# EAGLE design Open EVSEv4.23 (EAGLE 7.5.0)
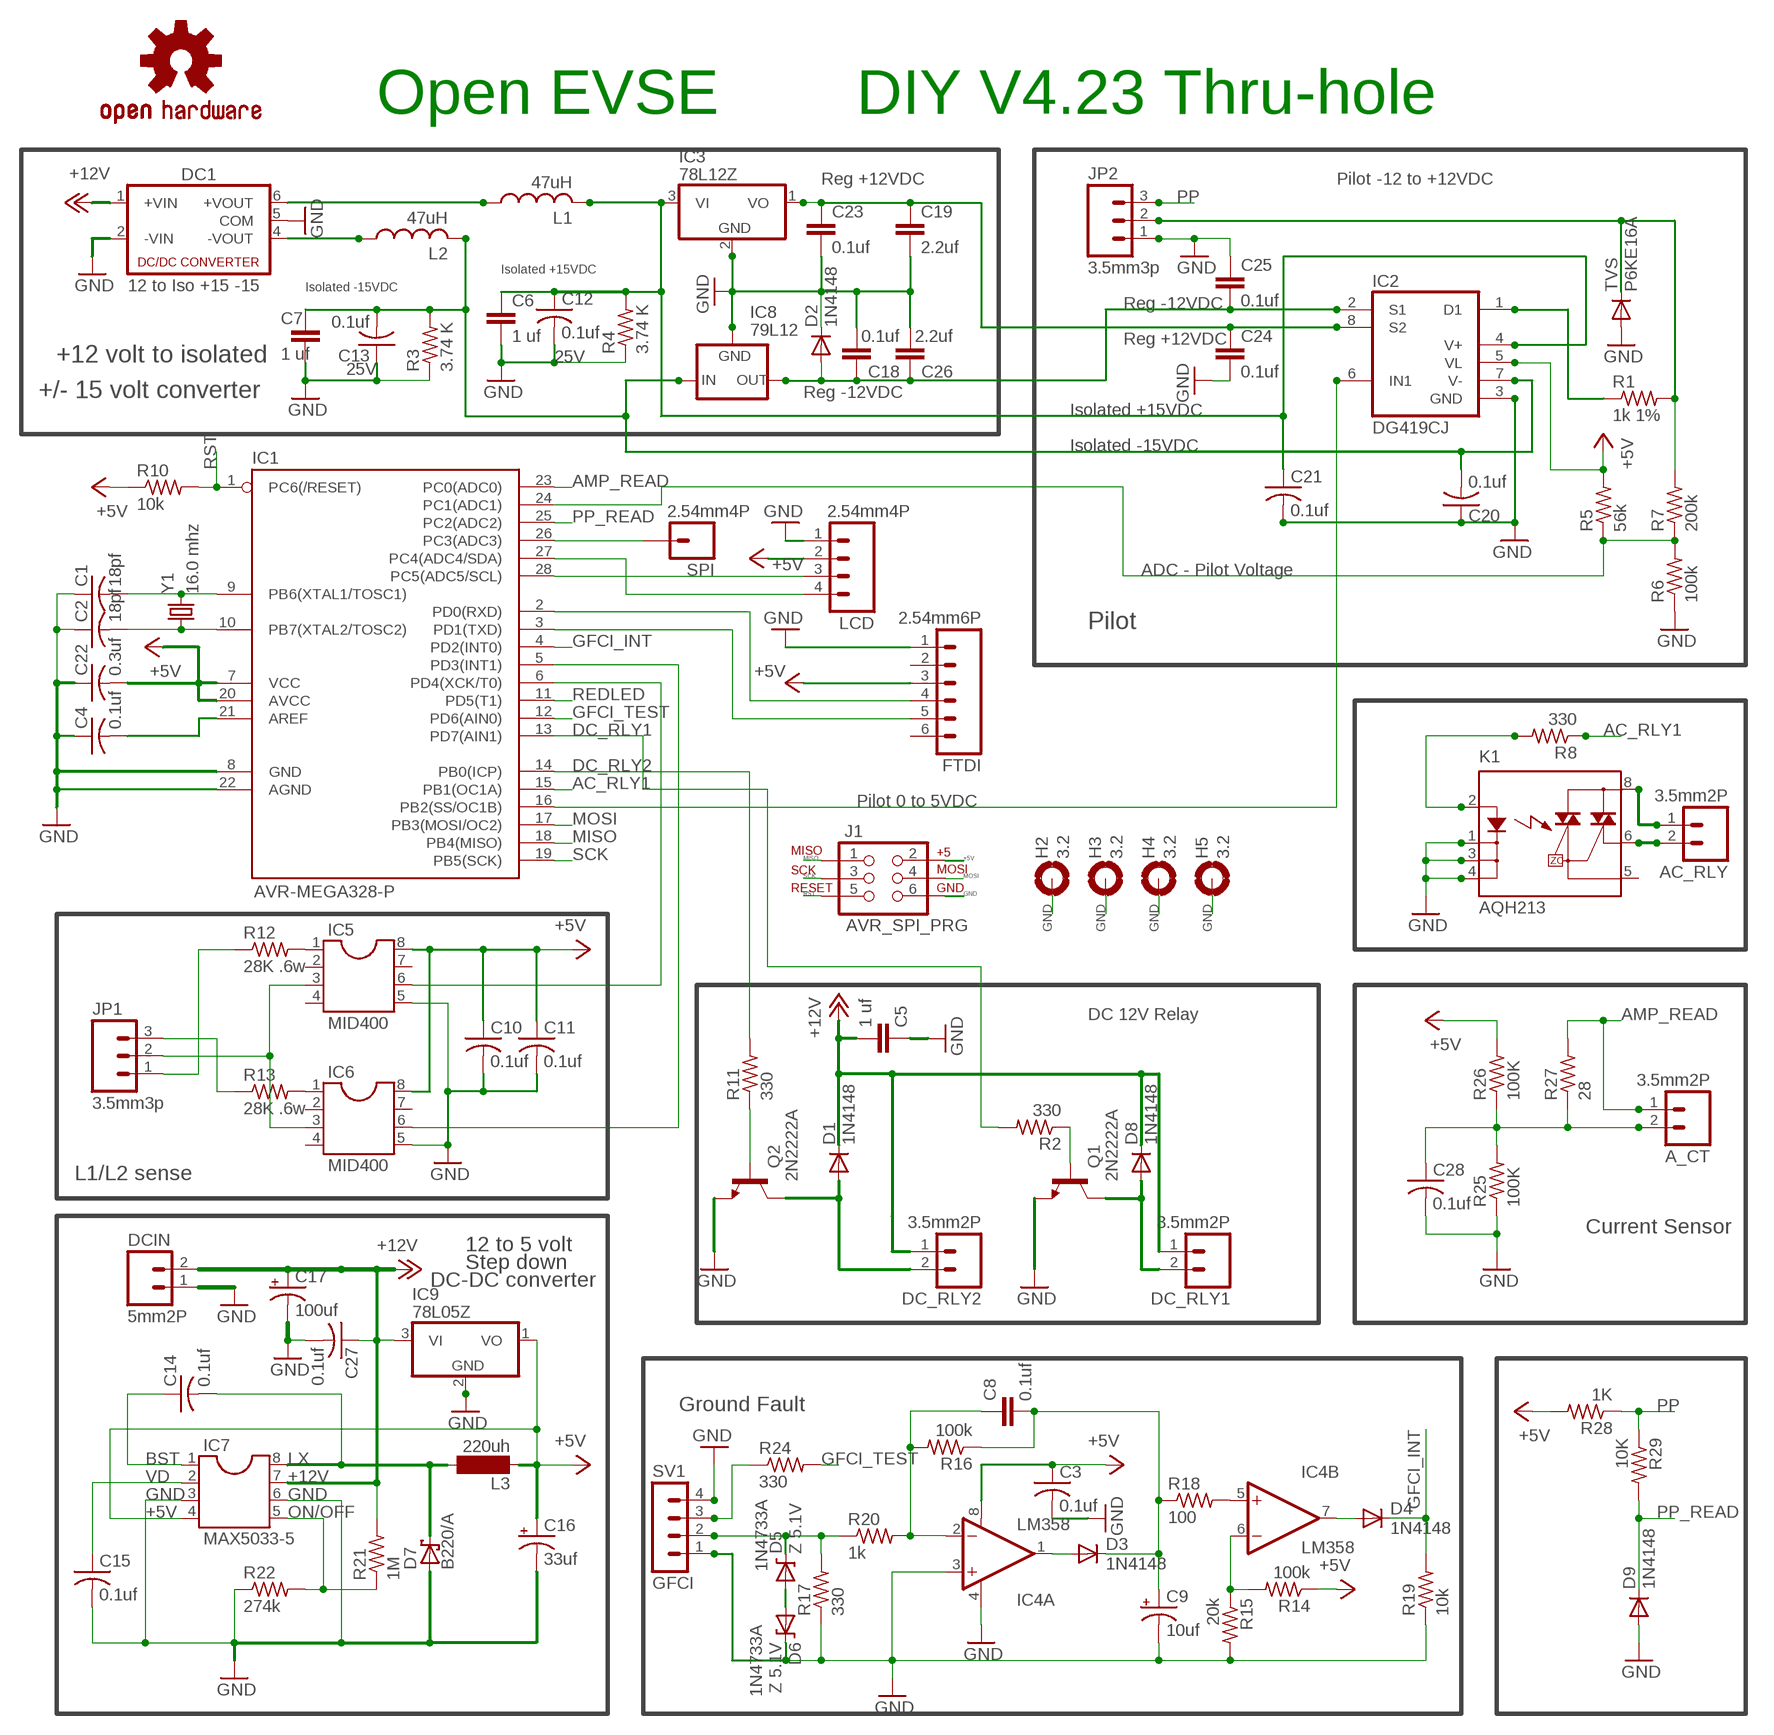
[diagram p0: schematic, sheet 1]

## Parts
A_CT  3.5mm2P  M023.5MM_LOCK  [SCREWTERMINAL-3.5MM-2_LOCK]
AC_RLY  3.5mm2P  M023.5MM_LOCK  [SCREWTERMINAL-3.5MM-2_LOCK]
C1  18pf  C-US025-024X044  [C025-024X044]
C2  18pf  C-US025-024X044  [C025-024X044]
C3  0.1uf  C-US025-025X050  [C025-025X050]
C4  0.1uf  C-US025-024X044  [C025-024X044]
C5  1 uf  CAPPTH  [CAP-PTH-SMALL]
C6  1 uf  CAPPTH  [CAP-PTH-SMALL]
C7  1 uf  CAPPTH  [CAP-PTH-SMALL]
C8  0.1uf  CAPEZ  [CAP-PTH-SMALLEZ]
C9  10uf  CAP_POLPTH2  [CPOL-RADIAL-10UF-25V]
C10  0.1uf  C-US025-025X050  [C025-025X050]
C11  0.1uf  C-US025-025X050  [C025-025X050]
C12  0.1uf  C-US025-025X050  [C025-025X050]
C13  0.1uf  C-US025-025X050  [C025-025X050]
C14  0.1uf  C-US025-025X050  [C025-025X050]
C15  0.1uf  C-US025-025X050  [C025-025X050]
C16  33uf  CPOL-USE2.5-7  [E2,5-7]
C17  100uf  CPOL-USE2.5-7  [E2,5-7]
C18  0.1uf  CAPEZ  [CAP-PTH-SMALLEZ]
C19  2.2uf  CAPEZ  [CAP-PTH-SMALLEZ]
C20  0.1uf  C-US025-025X050  [C025-025X050]
C21  0.1uf  C-US025-025X050  [C025-025X050]
C22  0.3uf  C-US025-024X044  [C025-024X044]
C23  0.1uf  CAPEZ  [CAP-PTH-SMALLEZ]
C24  0.1uf  CAPPTH  [CAP-PTH-SMALL]
C25  0.1uf  CAPPTH  [CAP-PTH-SMALL]
C26  2.2uf  CAPEZ  [CAP-PTH-SMALLEZ]
C27  0.1uf  C-US025-025X050  [C025-025X050]
C28  0.1uf  C-US025-025X050  [C025-025X050]
D1  1N4148  DIODE1N4148  [DIODE-1N4148]
D2  1N4148  DIODE1N4148  [DIODE-1N4148]
D3  1N4148  DIODE1N4148  [DIODE-1N4148]
D4  1N4148  DIODE1N4148  [DIODE-1N4148]
D5  Z 5.1V  DIODE-ZENERPTH  [DIODE-ZENER]
D6  Z 5.1V  DIODE-ZENERPTH  [DIODE-ZENER]
D7  B220/A  SCHOTTKY-DIODEF126Z12  [F126Z12]
D8  1N4148  DIODE1N4148  [DIODE-1N4148]
D9  1N4148  DIODE1N4148  [DIODE-1N4148]
DC1  12 to Iso +15 -15  MEV1D  [NMA7]
DC_RLY1  3.5mm2P  M023.5MM_LOCK  [SCREWTERMINAL-3.5MM-2_LOCK]
DC_RLY2  3.5mm2P  M023.5MM_LOCK  [SCREWTERMINAL-3.5MM-2_LOCK]
DCIN  5mm2P  M025MM  [SCREWTERMINAL-5MM-2]
FTDI  2.54mm6P  M06LOCK  [1X06_LOCK]
H2  3.2  MOUNT-PAD-ROUND3.2  [3,2-PAD]
H3  3.2  MOUNT-PAD-ROUND3.2  [3,2-PAD]
H4  3.2  MOUNT-PAD-ROUND3.2  [3,2-PAD]
H5  3.2  MOUNT-PAD-ROUND3.2  [3,2-PAD]
IC1  AVR-MEGA328-P  AVR-MEGA8-PSIM  [DIL28-3-SIMON]
IC2  DG419CJ  [DIL08]
IC3  78L12Z  [TO92]
IC4  LM358  OPAMP-DUALDIP  [DIP08]
IC5  MID400  DIL8S  [SOCKET-08]
IC6  MID400  DIL8S  [SOCKET-08]
IC7  MAX5033-5  DIL8  [DIL08]
IC8  79L12  79LXX  [79LXX]
IC9  78L05Z  [TO92]
J1  AVR_SPI_PRG  AVR_SPI_PRG_6PTH  [2X3]
JP1  3.5mm3p  M03SCREW_LOCK  [SCREWTERMINAL-3.5MM-3_LOCK.007S]
JP2  3.5mm3p  M03SCREW_LOCK  [SCREWTERMINAL-3.5MM-3_LOCK.007S]
K1  AQH213  [DIL07]
L1  47uH  L-US0204V  [0204V]
L2  47uH  L-US0204V  [0204V]
L3  220uh  BS11  [BS11]
LCD  2.54mm4P  M04LOCK  [1X04_LOCK]
Q1  2N2222A  [TO18]
Q2  2N2222A  [TO18]
R1  1k 1%  R-US_0204/7  [0204/7]
R2  330  R-US_0204/7  [0204/7]
R3  3.74 K  R-US_0204/7  [0204/7]
R4  3.74 K  R-US_0204/7  [0204/7]
R5  56k  R-US_0204/7  [0204/7]
R6  100k  R-US_0204/7  [0204/7]
R7  200k  R-US_0204/7  [0204/7]
R8  330  R-US_0204/7  [0204/7]
R10  10k  R-US_0204/7  [0204/7]
R11  330  R-US_0204/7  [0204/7]
R12  28K .6w  R-US_0207/10  [0207/10]
R13  28K .6w  R-US_0207/10  [0207/10]
R14  100k  R-US_0204/7  [0204/7]
R15  20k  R-US_0204/7  [0204/7]
R16  100k  R-US_0204/7  [0204/7]
R17  330  R-US_0204/7  [0204/7]
R18  100  R-US_0204/7  [0204/7]
R19  10k  R-US_0204/7  [0204/7]
R20  1k  R-US_0204/7  [0204/7]
R21  1M  R-US_0204/7  [0204/7]
R22  274k  R-US_0204/7  [0204/7]
R24  330  R-US_0204/7  [0204/7]
R25  100K  R-US_0204/7  [0204/7]
R26  100K  R-US_0204/7  [0204/7]
R27  28  R-US_0204/7  [0204/7]
R28  1K  R-US_0204/7  [0204/7]
R29  10K  R-US_0204/7  [0204/7]
SPI  2.54mm4P  M01PTH  [1X01]
SV1  GFCI  MA04-1  [MA04-1]
TVS  P6KE16A  DIODEPTH  [DIODE-1N4001]
U$1  OSHW-LOGOL  [OSHW-LOGO-L]
Y1  16.0 mhz  CRYSTALHC49UV  [HC49U-V]

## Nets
+5V: C3.1 C10.1 C11.1 C16.+ C22.2 FTDI.3 IC1.7(VCC) IC1.20(AVCC) IC2.5(VL) IC4.8(A:V+) IC5.8 IC6.8 IC7.4 IC9.1(VO) J1.2 L3.1 LCD.2 R5.2 R10.1 R14.1 R26.2 R28.2
+12V: C5.1 C17.+ C27.1 D1.C D8.C DC1.1(+VIN) DC_RLY1.1 DC_RLY2.1 DCIN.2 IC7.7 IC9.3(VI) R21.2
+12VI: DC1.6(+VOUT) L1.1
+12VIF: C6.1 C12.1 C21.1 IC2.4(V+) IC3.3(VI) L1.2 R4.2
-12VI: DC1.4(-VOUT) L2.1
-12VIF: C7.1 C13.2 C20.2 IC2.7(V-) IC8.IN L2.2 R3.2
AC_RLY1: IC1.15(PB1(OC1A)) R8.1
AMP_READ: A_CT.1 IC1.23(PC0(ADC0)) R27.2
BST: C14.1 IC7.1
DC_RLY1: IC1.13(PD7(AIN1)) R2.2
DC_RLY2: IC1.14(PB0(ICP)) R11.2
GFCI_INT: D4.C IC1.4(PD2(INT0)) R19.2
GFCI_TEST: IC1.12(PD6(AIN0)) R24.2
GND: C1.1 C2.1 C3.2 C4.1 C5.2 C6.2 C7.2 C9.2(-) C10.2 C11.2 C12.2 C13.1 C15.2 C16.- C17.- C18.2 C19.2 C20.1 C21.2 C22.1 C23.2 C24.2 C25.1 C26.2 C27.2 C28.2 D2.C D6.P$1(C) D7.A D9.A DC1.2(-VIN) DC1.5(COM) DCIN.1 FTDI.1 H2.B3,2(MOUNT) H3.B3,2(MOUNT) H4.B3,2(MOUNT) H5.B3,2(MOUNT) IC1.8(GND) IC1.22(AGND) IC2.3(GND) IC3.2(GND) IC4.3(A:+IN) IC4.4(A:V-) IC5.5 IC6.5 IC7.3 IC7.6 IC8.GND IC9.2(GND) J1.6 JP2.1 K1.1(K) K1.3(K1) K1.4(K2) LCD.1 Q1.1(E) Q2.1(E) R3.1 R4.1 R6.1 R15.2 R17.1 R19.1 R22.1 R25.1 SV1.1 SV1.4 TVS.A
LX: C14.2 D7.C IC7.8 L3.2
MISO: IC1.18(PB4(MISO)) J1.1
MOSI: IC1.17(PB3(MOSI/OC2)) J1.4
N$1: IC1.28(PC5(ADC5/SCL)) LCD.3
N$2: Q2.2(B) R11.1
N$3: JP1.3 R13.1
N$4: C1.2 IC1.9(PB6(XTAL1/TOSC1)) Y1.2
N$5: C2.2 IC1.10(PB7(XTAL2/TOSC2)) Y1.1
N$6: IC1.27(PC4(ADC4/SDA)) LCD.4
N$7: C4.2 IC1.21(AREF)
N$8: FTDI.5 IC1.3(PD1(TXD))
N$9: Q1.2(B) R2.1
N$10: IC2.1(D1) R1.1
N$11: R24.1 SV1.3
N$12: FTDI.4 IC1.2(PD0(RXD))
N$13: D1.A DC_RLY2.2 Q2.3(C)
N$14: K1.2(A) R8.2
N$15: C19.1 C23.1 C24.1 IC2.8(S2) IC3.1(VO)
N$16: C18.1 C25.2 C26.1 D2.A IC2.2(S1) IC8.OUT
N$17: JP1.1 R12.1
N$18: C8.1 IC4.2(A:-IN) R16.2 R20.2
N$19: IC4.5(B:+IN) R18.2
N$20: D5.P$1(C) R17.2 R20.1 SV1.2
N$21: D3.A IC4.1(A:OUT)
N$22: D5.P$2(A) D6.P$2(A)
N$23: C8.2 C9.1(+) D3.C R16.1 R18.1
N$24: IC4.6(B:-IN) R14.2 R15.1
N$25: D4.A IC4.7(B:OUT)
N$26: IC1.26(PC3(ADC3)) SPI.1
N$27: D8.A DC_RLY1.2 Q1.3(C)
N$29: IC1.6(PD4(XCK/T0)) IC5.6
N$30: IC1.5(PD3(INT1)) IC6.6
N$31: AC_RLY.2 K1.6(DS3)
N$33: A_CT.2 C28.1 R25.2 R26.1 R27.1
N$34: AC_RLY.1 K1.8(DS1)
N$37: JP2.2 R1.2 R7.2 TVS.C
N$39: IC5.1 R12.2
N$42: IC6.1 R13.2
N$43: IC5.3 IC6.3 JP1.2
N$53: IC1.24(PC1(ADC1)) R5.1 R6.2 R7.1
ON/OFF: IC7.5 R21.1 R22.2
PILOT: IC1.16(PB2(SS/OC1B)) IC2.6(IN1)
PP: JP2.3 R28.1 R29.1
PP_READ: D9.C IC1.25(PC2(ADC2)) R29.2
REDLED: IC1.11(PD5(T1))
RST: IC1.1(PC6(/RESET)) J1.5 R10.2
SCK: IC1.19(PB5(SCK)) J1.3
VD: C15.1 IC7.2
Unconnected: FTDI.2 FTDI.6 IC5.2 IC5.4 IC5.7 IC6.2 IC6.4 IC6.7 K1.5(DS2)

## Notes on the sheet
- Open EVSE | DIY V4.23 Thru-hole
- Reg +12VDC | Pilot -12 to +12VDC
- Isolated +15VDC
- Isolated -15VDC
- Reg -12VDC
- Reg +12VDC
- +12 volt to isolated
- +/- 15 volt converter | Reg -12VDC
- Isolated +15VDC
- Isolated -15VDC
- ADC - Pilot Voltage
- Pilot
- DC_RLY2
- Pilot 0 to 5VDC
- DC 12V Relay
- L1/L2 sense
- Current Sensor
- 12 to 5 volt
- Step down
- DC-DC converter
- Ground Fault

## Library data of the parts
A_CT AC_RLY DC_RLY1 DC_RLY2 DCIN = SparkFun:M02: Header 2
C1 C2 C4 C22 = adafruit:C-US: CAPACITOR, American symbol
C3 C10 C11 C14 C15 C20 C21 C27 C28 = resistor:C-US: CAPACITOR, American symbol
C5-C8 = SparkFun-Capacitors:CAP: Capacitor
C9 = SparkFun:CAP_POL: Capacitor Polarized
C12 C13 = resistor:C-US: CAPACITOR, American symbol; VOLTAGE: 25V
C16 C17 = resistor:CPOL-US: POLARIZED CAPACITOR, American symbol
C18 C19 C23-C26 = SparkFun-Passives:CAP: Capacitor
D1 D3 D4 D8 D9 TVS = SparkFun:DIODE: Diode
D2 = SparkFun-DiscreteSemi:DIODE: Diode
D5 D6 = SparkFun:DIODE-ZENER: Zener Diode; TYPE: 1N4733A
D7 = diode:SCHOTTKY-DIODE: Schottky Diode
DC1 = dc-dc-converter2:MEV1D: muRata MEV1DXXXXSC DC-DC converter isolated output 5 pin wide spacing 3,4 not populated
FTDI = SparkFun:M06: Header 6 Standard 6-pin 0.1" header. Use with straight break away headers (SKU : PRT-00116), right angle break away headers (PRT-00553), swiss pins (PRT-00743), machine pins (PRT-00117), and female headers (PRT-00115). Molex polarized connector foot print use with SKU : PRT-08094 with associated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
H2-H5 = holes:MOUNT-PAD-ROUND: MOUNTING PAD, round
IC1 = SparkFun:AVR-MEGA8-P: MICROCONTROLLER 8 Kbytes FLASH 1 kbytes SRAM 512 bytes EEPROM USART 4-channel 10 bit ADC 2-channel 8 bit ADC
IC2 = maxim:DG419CJ: ANALOG SWITCH; MF: MAXIM; MPN: DG419CJ; OC_FARNELL: unknown; OC_NEWARK: 77C6520
IC3 IC9 = linear:78*: Positive VOLTAGE REGULATOR Source: http://cache.national.com/ds/LM/LM78L05.pdf http://www.fairchildsemi.com/ds/LM/LM7805.pdf
IC4 = SparkFun:OPAMP-DUAL: Operational Amplifier
IC5-IC7 = ic-package:DIL8: Dual In Line / Socket
IC8 = v-reg:79LXX: VOLTAGE REGULATOR
J1 = SparkFun:AVR_SPI_PRG_6: AVR ISP 6 Pin This is the reduced ISP connector for AVR programming. Common on Arduino. This footprint will take up less PCB space and can be used with a 10-pin to 6-pin adapter such as SKU: BOB-08508
JP1 JP2 = SparkFun:M03: Header 3 Standard 3-pin 0.1" header. Use with straight break away headers (SKU : PRT-00116), right angle break away headers (PRT-00553), swiss pins (PRT-00743), machine pins (PRT-00117), and female headers (PRT-00115). Molex polarized connector foot print use with SKU : PRT-08232 with associated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
K1 = relay:AQH*213: SOLID STATE RELAY NAiS Source: http://www.mew-europe.com/.. en_ds_61613_0000.pdf; OC_FARNELL: unknown; OC_NEWARK: unknown
L1 L2 = resistor:L-US: INDUCTOR, American symbol
L3 = inductor-neosid:BS: INDUCTOR; OC_FARNELL: unknown; OC_NEWARK: unknown
LCD = SparkFun:M04: Header 4 Standard 4-pin 0.1" header. Use with straight break away headers (SKU : PRT-00116), right angle break away headers (PRT-00553), swiss pins (PRT-00743), machine pins (PRT-00117), and female headers (PRT-00115). Molex polarized connector foot print use with SKU : PRT-08231 with associated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
Q1 Q2 = transistor-npn:2N2222*: NPN Transistor
R1 R2 R5-R8 R10 R11 R14-R20 R24-R29 = adafruit:R-US_: RESISTOR, American symbol
R3 R4 R12 R13 R21 R22 = resistor:R-US_: RESISTOR, American symbol
SPI = SparkFun-Connectors:M01: Header 1
SV1 = con-lstb:MA04-1: PIN HEADER; OC_FARNELL: unknown; OC_NEWARK: unknown
U$1 = SparkFun-Aesthetics:OSHW-LOGO: Open Source Hardware Logo This logo indicates the piece of hardware it is found on incorporates a OSHW license and/or adheres to the definition of open source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
Y1 = SparkFun:CRYSTAL: Crystals

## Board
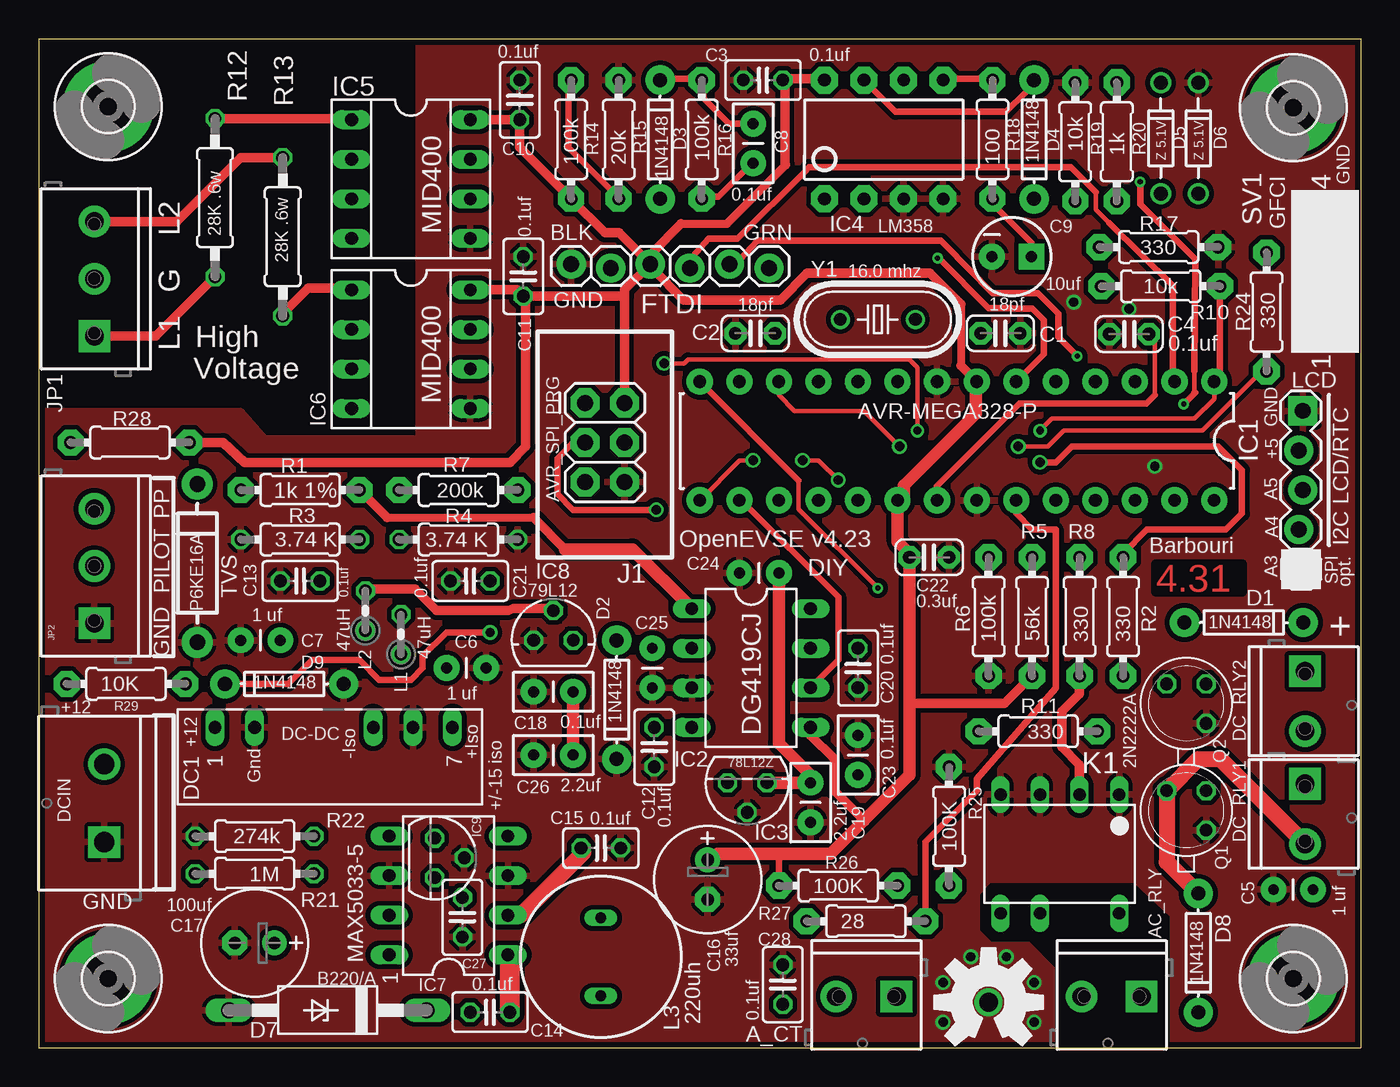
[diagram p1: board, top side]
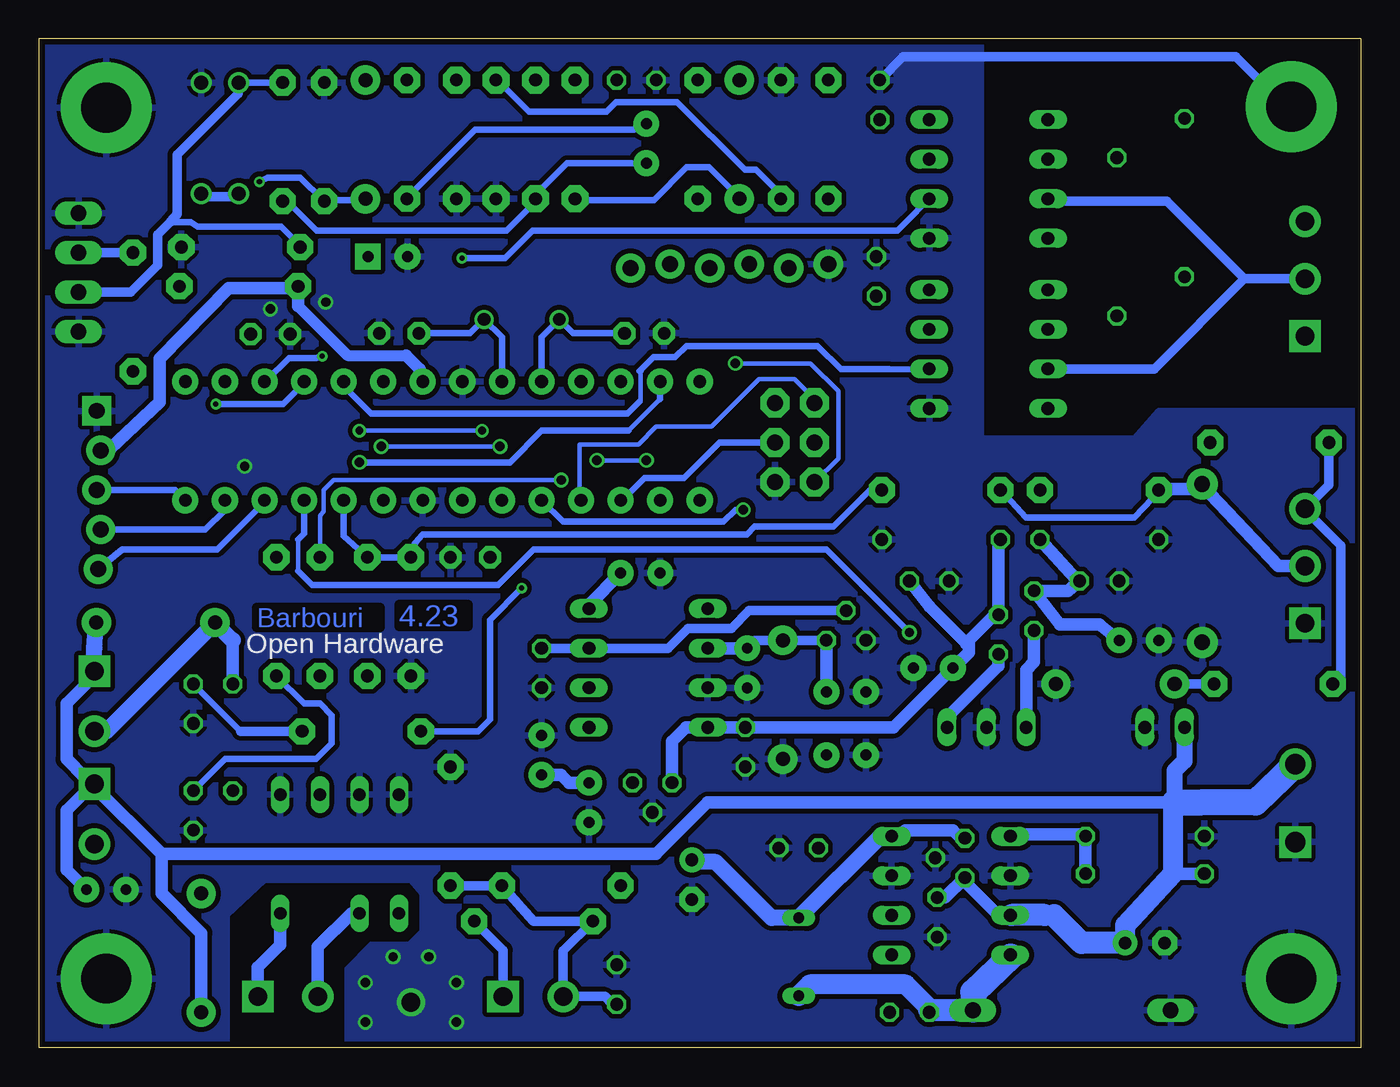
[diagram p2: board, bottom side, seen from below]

Size 84.84 x 64.77 mm. Coordinates in mm from the lower left corner, seen from the top.
Outline: 0,0 84.84,0 84.84,64.77 0,64.77 0,0
Copper layers (1*16): Top 0.0356mm / dielectric 1.5011mm / Bottom 0.0356mm
Design rules "default *": minimum track width 6mil, minimum drill 13mil, track to track 12mil, track to pad 12mil, pad to pad 12mil, via to via 12mil, smd to smd 6mil, copper to edge 15mil, drill to drill 6mil, minimum pad ring 7mil, minimum via ring 7mil, stop-mask expansion 4mil, vias tented up to drill 0mil, thermal gap 10mil

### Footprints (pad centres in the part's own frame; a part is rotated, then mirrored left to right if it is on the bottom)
SCREWTERMINAL-3.5MM-2_LOCK = drill 1.2 pad 2.032 square: 1 -0.178,0 | drill 1.2 pad 2.032: 2 3.678,0
C025-024X044 = drill 0.813 pad 1.422 octagon: 1 -1.27,0; 2 1.27,0
C025-025X050 = drill 0.813 octagon: 1 -1.27,0; 2 1.27,0
CAP-PTH-SMALL = drill 0.7 pad 1.651: 1 0,0; 2 2.54,0
CAP-PTH-SMALLEZ = drill 0.7 pad 1.651: 1 0,0; 2 2.54,0
CPOL-RADIAL-10UF-25V = drill 0.7 pad 1.651 square: 1 1.27,0 | drill 0.7 pad 1.651: 2 -1.27,0
E2,5-7 = drill 0.813 pad 1.6: + -1.27,0 | drill 0.813 pad 1.6 octagon: - 1.27,0
DIODE-1N4148 = drill 0.9 pad 1.88: A -3.81,0; C 3.81,0
DIODE-ZENER = drill 0.9: P$1 -3.556,0; P$2 3.556,0
F126Z12 = drill 1.016 long: A 6.35,0; C -6.35,0
NMA7 = drill 0.813 long: 1 1.27,7.62; 2 1.27,5.08; 4 1.27,-2.54; 5 1.27,-5.08; 6 1.27,-7.62
SCREWTERMINAL-5MM-2 = drill 1.3 pad 2.032 square: 1 0,0 | drill 1.3 pad 2.032: 2 5,0
1X06_LOCK = drill 1.016 pad 1.88: 1 0,0; 2 2.54,-0.254; 3 5.08,0; 4 7.62,-0.254; 5 10.16,0; 6 12.7,-0.254
3,2-PAD = drill 3.2 pad 5.842: B3,2 0,0
DIL28-3-SIMON = drill 0.813 pad 1.676: 1 -16.51,-3.81; 2 -13.97,-3.81; 3 -11.43,-3.81; 4 -8.89,-3.81; 5 -6.35,-3.81; 6 -3.81,-3.81; 7 -1.27,-3.81; 8 1.27,-3.81; 9 3.81,-3.81; 10 6.35,-3.81; 11 8.89,-3.81; 12 11.43,-3.81; 13 13.97,-3.81; 14 16.51,-3.81; 15 16.51,3.81; 16 13.97,3.81; 17 11.43,3.81; 18 8.89,3.81; 19 6.35,3.81; 20 3.81,3.81; 21 1.27,3.81; 22 -1.27,3.81; 23 -3.81,3.81; 24 -6.35,3.81; 25 -8.89,3.81; 26 -11.43,3.81; 27 -13.97,3.81; 28 -16.51,3.81
DIL08 = drill 0.813 long: 1 -3.81,-3.81; 2 -1.27,-3.81; 3 1.27,-3.81; 4 3.81,-3.81; 5 3.81,3.81; 6 1.27,3.81; 7 -1.27,3.81; 8 -3.81,3.81
TO92 = drill 0.813 octagon: 1 -1.27,0; 2 0,1.905; 3 1.27,0
DIP08 = drill 0.813 pad 1.727 octagon: 1 -3.81,-3.81; 2 -1.27,-3.81; 3 1.27,-3.81; 4 3.81,-3.81; 5 3.81,3.81; 6 1.27,3.81; 7 -1.27,3.81; 8 -3.81,3.81
SOCKET-08 = drill 0.813 long: 1 -3.81,-3.81; 2 -1.27,-3.81; 3 1.27,-3.81; 4 3.81,-3.81; 5 3.81,3.81; 6 1.27,3.81; 7 -1.27,3.81; 8 -3.81,3.81
79LXX = drill 0.813 octagon: GND -1.27,0; IN 0,1.905; OUT 1.27,0
2X3 = drill 1.016 pad 1.88 octagon: 1 0,0; 2 0,2.54; 3 2.54,0; 4 2.54,2.54; 5 5.08,0; 6 5.08,2.54
SCREWTERMINAL-3.5MM-3_LOCK.007S = drill 1.2 pad 2.032 square: 1 -0.178,0 | drill 1.2 pad 2.032: 2 3.5,0; 3 7.178,0
DIL07 = drill 0.8 long: 1 -3.81,-3.81; 2 -1.27,-3.81; 3 1.27,-3.81; 4 3.81,-3.81; 5 3.81,3.81; 6 1.27,3.81; 8 -3.81,3.81
0204V = drill 0.813 octagon: 1 -1.27,0; 2 1.27,0
BS11 = drill 0.7 long: 1 -2.5,0; 2 2.5,0
1X04_LOCK = drill 1.016 pad 1.88 square: 1 0,0.127 | drill 1.016 pad 1.88: 2 2.54,-0.127; 3 5.08,0.127; 4 7.62,-0.127
TO18 = drill 0.813 octagon: 1 -1.27,-1.27; 2 1.27,-1.27; 3 1.27,1.27
0204/7 = drill 0.813 pad 1.676 octagon: 1 -3.81,0; 2 3.81,0
0204/7' = drill 0.813 octagon: 1 -3.81,0; 2 3.81,0
0207/10 = drill 0.813 octagon: 1 -5.08,0; 2 5.08,0
1X01 = drill 1.016 pad 1.88: 1 0,0
MA04-1 = drill 1.016 long: 1 -3.81,0; 2 -1.27,0; 3 1.27,0; 4 3.81,0
DIODE-1N4001 = drill 1 pad 1.981: A -5.08,0; C 5.08,0
HC49U-V = drill 0.813: 1 -2.413,0; 2 2.413,0

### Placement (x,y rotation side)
A_CT  54.86,3.3 180 top
AC_RLY  70.61,3.3 180 top
C1  61.72,45.87 180 top
C2  45.97,45.87 0 top
C3  46.48,62.13 180 top
C4  69.98,45.82 0 top
C5  81.79,10.16 180 top
C6  26.16,24.38 0 top
C7  15.49,26.16 180 top
C8  45.85,56.79 90 top
C9  62.45,50.8 0 top
C10  30.86,60.86 90 top
C11  31.09,49.53 90 top
C12  39.5,19.3 270 top
C13  16.76,29.97 0 top
C14  28.96,2.29 180 top
C15  36.07,12.83 0 top
C16  42.93,10.79 270 top
C17  13.84,6.73 180 top
C18  34.29,22.86 180 top
C19  49.53,17.02 270 top
C20  52.58,24.38 90 top
C21  27.69,29.97 180 top
C22  57.15,31.5 180 top
C23  52.58,17.53 90 top
C24  47.5,30.48 180 top
C25  39.37,23.11 90 top
C26  34.29,18.8 180 top
C27  27.18,8.38 270 top
C28  47.75,4.06 90 top
D1  77.34,27.3 0 top
D2  37.08,22.35 270 top
D3  39.88,58.32 90 top
D4  63.88,58.32 270 top
D5  72.01,58.39 270 top
D6  74.42,58.39 270 top
D7  18.54,2.41 180 top
D8  74.42,6.1 270 top
D9  15.75,23.37 180 top
DC1  18.92,19.3 90 top
DC_RLY1  81.28,16.76 270 top
DC_RLY2  81.28,24 270 top
DCIN  4.19,13.21 90 top
FTDI  34.16,50.32 0 top
H2  4.45,60.43 0 top
H3  4.45,4.45 0 top
H4  80.52,4.45 0 top
H5  80.52,60.35 0 top
IC1  58.93,38.96 180 top
IC2  45.72,24.38 270 top
IC3  45.47,17.02 180 top
IC4  54.23,58.32 0 top
IC5  23.88,55.78 270 top
IC6  23.88,44.86 270 top
IC7  26.29,9.78 90 top
IC8  33.02,26.16 0 top
IC9  25.4,12.19 270 top
J1  35.05,41.4 270 top
JP1  3.56,45.87 90 top
JP2  3.56,27.43 90 top
K1  65.53,12.45 180 top
L1  23.24,26.54 90 top
L2  20.96,28.07 90 top
L3  36.07,5.84 270 top
LCD  81,40.89 270 top
Q1  73.66,15.24 90 top
Q2  73.66,22.1 90 top
R1  16.76,35.81 180 top
R2  69.6,27.69 90 top
R3  3.74 K  [0204/7']  16.76,32.64 0 top
R4  3.74 K  [0204/7']  26.92,32.64 180 top
R5  63.75,27.69 270 top
R6  60.96,27.69 90 top
R7  26.92,35.81 180 top
R8  66.8,27.69 270 top
R10  72.01,48.9 0 top
R11  64.13,20.32 180 top
R12  11.3,54.58 90 top
R13  15.65,52.07 270 top
R14  34.16,58.32 90 top
R15  37.21,58.32 90 top
R16  42.55,58.32 270 top
R17  71.88,51.41 180 top
R18  61.21,58.32 90 top
R19  66.52,58.17 270 top
R20  69.19,58.17 270 top
R21  1M  [0204/7']  13.84,11.18 180 top
R22  274k  [0204/7']  13.84,13.59 0 top
R24  78.8,47.24 270 top
R25  58.42,14.22 270 top
R26  51.31,10.41 180 top
R27  53.09,8.13 0 top
R28  5.84,38.86 0 top
R29  5.59,23.37 0 top
SPI  81.03,30.73 0 top
SV1  82.3,49.78 90 top
TVS  10.16,31.11 90 top
U$1  60.96,2.92 0 top
Y1  53.85,46.76 0 top

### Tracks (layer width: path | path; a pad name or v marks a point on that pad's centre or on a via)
+5V
  Top 0.406: 47.9,62.23 47.88,62.23 | 39.34,50.49 FTDI.3 | 55.17,35.2 IC1.20 | 60.15,42.67 IC1.7 | R26.2 47.5,12.45
  Top 0.508: 47.9,56.67 47.95,56.72 47.95,56.69 44.17,52.91 41.22,52.91 | 47.9,61.8 47.9,62.23 | 59.18,47.75 59.18,43.79
  Top 0.61: 47.9,62.23 50.37,62.23 IC4.8 | 47.88,62.23 C3.1 | 47.9,56.67 47.9,61.8 | 41.22,52.91 39.34,51.03 39.34,50.49 | FTDI.3 39.34,50.06 41.38,48.01 47.59,48.01 49.31,49.73 57.2,49.73 59.18,47.75 | IC5.8 C10.1 30.86,57.81 R14.1 34.16,54.48 36.32,52.32 37.24,52.32 FTDI.3 | J1.2 37.59,48.26 | 37.59,48.26 37.59,48.67 FTDI.3 | C11.1 37.59,48.26 | 59.18,43.79 IC1.7 | IC2.5 49.53,20.07 51.05,18.54 51.05,16.51 52.96,14.61 | R5.2 61.98,22.1 55.88,22.1 | IC6.8 30.68,48.67 C11.1 | R28.2 11.81,38.86 13.21,37.59 30.23,37.59 31.24,38.61 31.24,48.11 C11.1
  Top 0.813: 55.17,35.2 55.52,35.56 55.52,36.09 60.15,40.72 60.15,42.67 | IC1.20 55.12,32.51 55.88,31.75 C22.2 55.88,22.1 55.88,17.53 52.96,14.61 50.8,12.45 47.5,12.45 43.56,12.45 C16.+
  Bottom 0.61: 60.4,42.98 IC1.7 | LCD.2 80.26,38.48 | 68.33,48.77 R10.1
  Bottom 0.711: 68.2,47.62 65.02,44.45 61.28,44.45
  Bottom 0.813: R10.1 68.2,47.62 | 61.28,44.45 60.4,43.57 60.4,42.98 | 42.8,11.94 C16.+ | IC9.1 25.65,13.46 26.16,13.97 29.21,13.97 29.46,13.72 29.97,13.72 IC7.4 | 80.26,38.48 77.09,41.47 77.09,44.26 72.64,48.77 68.33,48.77
  Bottom 1.016: IC7.4 30.82,13.59 L3.1 37.81,8.34 41.4,11.94 42.8,11.94
+12V
  Bottom 0.406: 22.4,8.53 IC7.7 | DC_RLY1.1 81.92,16.94 81.92,17.4
  Bottom 0.813: 12.07,11.18 R21.2 | 12.07,15.62 10.29,15.75 | 81.28,23.88 83.06,22.1 83.06,18.54 81.92,17.4 81.41,16.89 | 81.41,16.89 76.96,12.45 | 76.96,12.45 45.21,12.45 41.91,15.75 11.94,15.75 | DC_RLY2.1 81.28,24.13 | 81.41,16.89 83.06,15.24 83.06,11.43 C5.1 | D8.C 74.42,7.37 76.96,9.91 76.96,12.45 | IC7.7 22.61,8.38 23.11,8.38 25.4,10.67 IC9.3 26.67,9.65 C27.1
  Bottom 1.016: 81.28,23.88 81.28,24.13 81.28,25.65 D1.C | DC1.1 11.3,18.41 11.94,17.78 11.94,15.75
  Bottom 1.27: 12.07,15.62 12.07,11.18 15.11,7.87 C17.+ | 20.27,8.53 19.68,8.51
  Bottom 1.422: C17.+ 17.91,6.73 19.68,8.51 | 20.27,8.53 22.4,8.53
  Bottom 1.676: DCIN.2 6.73,15.75 10.29,15.75 11.94,15.75
+12VI
  Bottom 0.813: L1.1 23.24,24.51 26.67,21.08 26.67,20.7 DC1.6
+12VIF
  Bottom 0.813: 25.3,25.96 25.15,25.96 25.15,25.4 C6.1 29.97,20.57 C12.1 IC2.4 43.31,20.57 44.2,19.68 IC3.3 | 25.3,25.96 25.32,25.96 23.5,27.79 L1.2 23.24,32.51 R4.2 | C21.1 27.69,28.35 25.3,25.96
-12VI
  Bottom 0.813: DC1.4 21.46,24.26 20.96,24.77 L2.1
-12VIF
  Top 0.61: L2.2 21.08,29.46 24.13,29.46 25.53,28.07 30.1,28.07 30.48,28.19 32.89,28.19 IC8.IN
  Bottom 0.61: IC8.IN 39.24,28.07 40.39,26.92 43.18,26.92 44.45,25.65 IC2.7 C20.2
  Bottom 0.813: C7.1 16.76,27.18 19.3,27.18 L2.2 18.8,29.34 C13.2 18.29,30.1 R3.2
AC_RLY1  (via drill 0.6)
  Top 0.305: v51.31,36.45 50.04,37.72 v49.02,37.72 | v45.85,37.72 44.98,37.72 IC1.15
  Bottom 0.305: R8.1 66.8,34.16 66.55,34.42 66.55,35.81 65.91,36.45 v51.31,36.45 | v49.02,37.72 v45.85,37.72
AMP_READ
  Top 0.406: IC1.23 62.74,34.29 63.75,33.27 65.28,33.27 65.28,23.11 60.2,17.27 60.2,16.51 56.9,13.21 R27.2
  Bottom 0.61: A_CT.1 55.04,6.27 R27.2
BST
  Top 0.813: 30.23,5.84 IC7.1
  Top 1.27: C14.1 30.23,5.84
DC_RLY1  (via drill 0.6)
  Top 0.406: R2.2 69.6,31.75 71.12,33.27 76.2,33.27 77.22,34.29 77.22,37.08 75.69,38.61 66.29,38.61 65.28,37.59 v64.26,37.59
  Bottom 0.305: 46.99,39.62 44.96,41.66
  Bottom 0.406: v64.26,37.59 54.61,37.59 52.58,39.62 46.99,39.62 | 44.96,41.66 IC1.13
DC_RLY2  (via drill 0.33)
  Top 0.305: 48.77,36.42 48.77,34.59 v53.85,29.52
  Top 0.406: 48.77,36.42 IC1.14
  Bottom 0.406: R11.2 56.64,20.32 55.88,21.08 55.88,27.48 v53.85,29.52
GFCI_INT  (via drill 0.33)
  Top 0.305: 74.17,43.43 74.17,42.06
  Top 0.406: v73.48,41.33 74.22,42.06 74.17,42.06 | 74.17,43.43 74.22,50.65 70.69,54.18 v70.69,55.6
  Bottom 0.406: v73.48,41.33 69.16,41.33 67.82,42.67 IC1.4 | v70.69,55.6 70.16,55.88 68.07,55.88 66.6,54.41 R19.2 66.45,54.41 64.01,54.41 D4.C
GFCI_TEST  (via drill 0.6)
  Top 0.305: R24.2 78.49,43.43 74.68,39.62 65.79,39.62 64.77,38.61 v62.87,38.61 | v55.24,38.61 52.96,40.89 48.51,40.89 47.5,41.91 IC1.12
  Bottom 0.305: v62.87,38.61 v55.24,38.61
GND  (via drill 0.6, 1.2)
  Bottom 0.61: H2.B3,2 4.8,60.43 8,63.63 29.36,63.63 C10.2
  other vias: 58.04,1.65 58.04,4.19 59.82,5.84 62.1,5.84 63.88,4.19 63.88,1.65 60.96,2.92 71.63,37.34 66.42,47.88 69.98,47.43
  pour Bottom: 0,0 65.02,0 65.02,5.08 63.5,6.6 61.09,6.6 60.2,7.49 60.2,9.91 60.96,10.79 70.36,10.79 72.77,8.51 72.77,0 84.84,0 84.84,64.77 24.38,64.77 24.38,39.12 14.48,39.12 12.95,40.89 0,40.89
  pour Top: 0,0 65.02,0 65.02,5.08 63.5,6.6 61.09,6.6 60.2,7.49 60.2,9.91 60.96,10.79 70.36,10.79 72.77,8.51 72.77,0 84.84,0 84.84,64.77 24.38,64.77 24.38,39.12 14.48,39.12 12.95,40.89 0,40.89
LX
  Bottom 0.61: 22.45,5.87 IC7.8
  Bottom 1.27: 24.87,2.46 D7.C | 27.69,2.41 C14.2 27.69,2.54 29.21,4.06 35.35,4.06 L3.2
  Bottom 1.422: D7.C 27.69,2.41
  Bottom 1.676: 24.87,2.46 24.87,3.58 22.45,5.87
MISO
  Bottom 0.305: J1.1 35.05,41.66 36.32,42.93 38.61,42.93 41.66,39.88 45.21,39.88 46.36,38.73 50.14,38.73 50.14,35.26 IC1.18
MOSI
  Bottom 0.406: IC1.17 47.35,35.2 45.97,36.58 43.43,36.58 41.15,38.86 J1.4 37.74,38.76
N$1
  Bottom 0.406: LCD.3 76.1,35.81 IC1.28
N$2
  Bottom 0.406: 71.88,20.32 Q2.2
  Bottom 0.61: R11.1 71.88,20.32
N$3
  Top 0.61: JP1.3 8.85,53.05 12.95,57.15 R13.1
N$4
  Bottom 0.406: IC1.9 55.12,45.62 Y1.2 57.15,45.87 C1.2
N$5
  Bottom 0.406: IC1.10 52.58,45.62 Y1.1 50.55,45.87 C2.2
N$6
  Bottom 0.406: LCD.4 74.17,33.27 72.9,34.54 IC1.27
N$7
  Top 0.305: 71.63,41.91 71.63,45.44
  Top 0.406: 57.66,35.2 IC1.21 57.66,36.07 62.69,41.1 62.94,41.38 71.09,41.38 71.63,41.91 | 71.63,45.44 C4.2
N$8  (via drill 0.33)
  Top 0.406: v66.65,44.4 65.43,45.62 65.43,47.14 64.11,48.46 61.21,48.46 58.17,51.56 57.91,51.82 46.13,51.82 44.6,50.19 FTDI.5
  Bottom 0.406: v66.65,44.4 67.06,44.3 68.78,44.3 70.26,42.82 IC1.3
N$9
  Bottom 0.406: Q1.2 72.9,18.54 67.06,18.54 66.04,19.56 66.04,21.34 66.8,22.1 67.82,22.1 R2.1
N$10
  Top 0.508: 22.35,34.04 31.75,34.04
  Top 0.61: R1.1 22.35,34.04 | 31.75,34.04 33.78,32
  Top 0.813: 33.78,32 38.1,32 IC2.1
N$11
  Bottom 0.61: SV1.3 R24.1
N$12
  Top 0.305: 68.71,52.96 67.86,53.81 67.86,54.94
  Top 0.406: 68.71,52.96 72.77,48.95 72.77,42.85 IC1.2 | 67.86,54.94 66.26,56.54 49.43,56.54 49.17,56.26 44.86,51.94 42.98,51.94 41.96,50.8 41.83,50.67 41.83,50.14 FTDI.4
N$13
  Bottom 0.813: 72.39,26.16 Q2.3 | DC_RLY2.2 80.51,20.32
  Bottom 1.016: 72.39,26.16 D1.A 80.51,20.32
N$14
  Top 0.61: K1.2 66.8,18.16 65.66,19.3 65.66,21.59 66.8,22.73 R8.2
N$15
  Top 0.813: C24.1 47.5,19.56 49.53,17.53 C19.1 IC3.1
  Bottom 0.813: IC2.8 49.53,28.45 C24.1 | C23.1 51.31,17.53 50.8,17.02 C19.1
N$16
  Top 0.813: C26.1 C18.1
  Bottom 0.61: IC8.OUT D2.A 38.86,26.16 C25.2
  Bottom 0.813: IC8.OUT C18.1 | C25.2 IC2.2
N$17
  Top 0.61: JP1.1 7.49,45.7 R12.1
N$18
  Top 0.406: C8.1 45.44,56.46 43.64,54.66 42.55,54.66 R16.2
  Bottom 0.406: C8.1 46.38,56.72 46.81,56.79 50.95,56.79 52.58,55.17 52.68,54.91 52.73,54.66 IC4.2 52.86,54.41 54.81,52.45 67,52.45 68.78,54.23 R20.2
N$19
  Top 0.406: R18.2 61.21,62.23 58.19,62.23 IC4.5
N$20
  Bottom 0.406: D5.P$1 71.7,61.87 71.53,61.95 69.65,61.95 69.22,61.87 R20.1 | 76.42,53.02 75.09,53.02 74.65,52.7 69.29,52.7 68.15,51.56 R17.2
  Bottom 0.61: D5.P$1 72.03,61.27 75.97,57.33 75.97,53.52 76.42,53.02 77.22,52.2 77.22,50.24 78.94,48.51 SV1.2
N$21
  Bottom 0.406: IC4.1 50.37,54.59 49.76,54.43 45.36,54.43 43.26,56.54 41.83,56.54 39.88,54.59 D3.A
N$22
  Bottom 0.61: D5.P$2 72.14,54.76 72.49,54.66 73.91,54.66 74.27,54.76 D6.P$2
N$23
  Top 0.406: C9.1 63.7,51.69 61.39,54 61.39,54.23 61.21,54.41 R18.1 | D3.C 39.88,62.23 42.37,62.23 R16.1 42.67,62 42.67,60.96 44.3,59.33 C8.2
  Bottom 0.406: R18.1 61.21,54.59 56.84,58.95 46.63,58.95 C8.2
N$24
  Top 0.406: R15.1 37.21,54.59 34.01,57.78 34.01,62.05 R14.2
  Bottom 0.406: IC4.6 55.35,62.05 53.39,60.1 48.41,60.1 47.8,60.71 43.87,60.71 39.52,56.36 38.81,56.36 37.21,54.76 37.21,54.59 R15.1
N$25
  Top 0.406: IC4.7 53.04,62.05 54.99,60.1 62.08,60.1 63.35,61.34 63.88,61.87 63.88,62.05 D4.A
N$26
  Bottom 0.406: IC1.26 70.36,35.05 73.41,32 79.5,32 SPI.1
N$27
  Top 1.016: D8.A 72.39,11.94 Q1.3 74.42,18.54 75.82,18.54 DC_RLY1.2
N$29  (via drill 0.33)
  Top 0.406: IC1.6 64.52,44.55 64.52,46.74 63.78,47.47 62.46,47.47 62.43,47.5 60.96,47.5 57.76,50.7 v57.68,50.7
  Bottom 0.406: v57.68,50.7 54.91,50.7 53.16,52.45 29.74,52.45 29.21,52.98 27.71,54.51 27.66,54.56 IC5.6
N$30
  Bottom 0.305: 46.28,41.5 46.23,41.63 46.23,43.43
  Bottom 0.406: 46.23,43.43 46.28,43.46 45.39,44.35 43.99,44.35 43.28,45.06 34.85,45.06 33.35,43.56 30.28,43.56 27.84,43.54 27.58,43.54 27.66,43.61 IC6.6 | 46.28,41.5 47.07,40.72 63.52,40.72 65.13,42.32 65.13,42.67 IC1.5
N$31
  Bottom 0.813: AC_RLY.2 66.93,6.47 64.77,8.64 K1.6
N$33
  Bottom 0.61: C28.1 48.01,2.79 48.51,3.3 A_CT.2 51.19,6.22 R27.1 53.09,8.13 R26.1 R25.2
N$34
  Bottom 0.813: AC_RLY.1 70.79,5.16 69.34,6.6 K1.8
N$37
  Bottom 0.406: 12.8,35.89 14.53,34.06 21.49,34.06 22.71,35.38 R7.2
  Bottom 0.61: 12.8,35.89 R1.2
  Bottom 0.813: 12.8,35.89 10.36,35.89 TVS.C 10.03,36.07 9.65,35.56 5.28,30.93 JP2.2
N$39
  Top 0.61: R12.2 19.99,59.66 IC5.1
N$42
  Top 0.61: R13.2 15.65,47.14 17.27,48.77 19.96,48.77 IC6.1
N$43
  Bottom 0.61: JP1.2 7.46,49.37 | 7.46,49.37 12.45,54.36 19.91,54.36 IC5.3 | IC6.3 13.25,43.59 7.46,49.37
N$53
  Bottom 0.406: IC1.24 65.28,32.87 R5.1 R6.2 60.71,32.41 60.2,32.97 39.37,32.97 38.91,33.48 33.83,33.48 31.5,35.81 R7.1
ON/OFF
  Bottom 0.406: IC7.5 22.55,13.56 22.45,13.69
  Bottom 0.61: 17.65,11.2 R21.1 | 17.65,13.51 R22.2 17.83,13.69
  Bottom 0.813: 17.65,13.51 17.65,11.2 | 17.83,13.69 22.45,13.69
PILOT
  Top 0.406: IC1.16 45.11,35.15 51.31,28.96 51.31,24.89 IC2.6
PP
  Bottom 0.61: R28.1 2.03,36.13 JP2.3 3.56,34.54 1.27,32.26 1.27,23.62 1.52,23.88 1.52,23.62 R29.1
PP_READ  (via drill 0.6)
  Top 0.406: v28.96,26.67 26.16,26.67 24.64,25.15 24.64,24.38 23.88,23.62 21.84,23.62 20.57,24.89 17.53,24.89 16,23.37 D9.C
  Bottom 0.305: 68.2,32.64 68.2,30.61
  Bottom 0.406: IC1.25 67.82,33.02 68.2,32.64 | 68.2,30.61 67.31,29.72 55.37,29.72 53.09,32 34.29,32 v28.96,26.67
  Bottom 0.61: R29.2 D9.C
RST  (via drill 0.5, 0.6)
  Top 0.305: v40.13,43.94 41.4,43.94 41.66,44.2 55.88,44.2 56.39,43.69 v56.39,39.62 | v64.26,39.62 65.02,40.39 74.17,40.39 75.44,41.66 IC1.1
  Top 0.406: IC1.1 75.44,42.85 75.79,43.2 75.79,48.9 R10.2
  Bottom 0.305: J1.5 33.53,37.85 33.53,42.16 35.31,43.94 v40.13,43.94 | v56.39,39.62 v64.26,39.62
SCK  (via drill 0.6)
  Top 0.406: v39.62,34.54 34.29,34.54 33.27,35.56 33.27,37.85 34.29,38.86 J1.3
  Bottom 0.406: IC1.19 51.21,33.78 40.89,33.78 40.13,34.54 v39.62,34.54
VD
  Top 0.813: 34.95,12.55 34.7,12.7 C15.1 | 30.94,8.53 IC7.2
  Top 1.016: 34.95,12.55 30.94,8.53

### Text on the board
Top: 4.31
Bottom: 4.23 | Barbouri
tPlace: I2C LCD/RTC | opt.
tNames: BLK | GRN | PP | PILOT | GND
_tsilk: GND | L2 | G | L1 | GND | High | Voltage | GND | +5 | A5 | A4 | OpenEVSE v4.23 | Barbouri | DIY | A3 | + | +12 | +12 | -Iso | +Iso | Gnd | +/-15 iso | GND | 1
_bsilk: Open Hardware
